| TEXAS INSTRUMENTS INCORPORATED
| Standard Linear and Logic Group
| IBIS Model of SN74AHCT16245
| 16-BIT BUS TRANSCEIVERS WITH 3-STATE OUTPUTS
| This file contains package information for the following:
|  SSOP 48-pin (DL) package as [Component] AHCT16245_DL
|  TSSOP 48-pin (DGG) package as [Component] AHCT16245_DGG
|  TVSOP 48-pin (DGV) package as [Component] AHCT16245_DGV
| This device can be powered at the following Vccs:
|  5 volt Vcc
| This file provides unique models under the [Model Selector] for each Vcc.
| For operation at a specific Vcc, select the appropriate model after each
| [Model Selector] keyword.
[IBIS Ver]   3.2
[Comment char]  |_char
[File Name]   sn74ahct16245.ibs
[File Rev]   1.1 | a_die
[Date]   January 15, 2001
[Source]   Data created from TI-SPICE simulations at TI-SLL.
[Notes]   The following is an IBIS list for the AHCT16245.
   Please contact sllibis@ti.com with questions and
   comments concerning SLL IBIS models.
[Disclaimer] Property of Texas Instruments Incorporated.  Unauthorized
   reproduction and/or distribution is strictly prohibited.
   This product is protected under copyright law.
   Created  2001, (C) Copyright  2001, Texas Instruments
   Incorporated, All Rights Reserved
   UNLESS THERE IS A SIGNED, WRITTEN AGREEMENT TO THE
   CONTRARY, TEXAS INSTRUMENTS (TI) IS PROVIDING THE IBIS
   MODELS  AND WITHOUT ANY WARRANTY, EXPRESSED OR
   IMPLIED.  TI assumes no liability for:
   1) the accuracy of the IBIS models provided to your
   company;
   2) the proper functioning of these IBIS Models in your
   design or for any resulting applications; or
   3) infringement of patents, copyrights or intellectual
   property rights resulting from your use of these IBIS
   models.
   TI provides IBIS Models as a service to our customers.
   You and your company shall not distribute, sell or give
   these models to anyone else without prior written
   permission from TI.
   TI reserves the right to make changes to our products or
   to discontinue any semiconductor product or service
   without notice, and advises our customers to obtain the
   latest version of relevant information to verify, before
   placing orders, that the information being relied on is
   current.
   Please be aware that your receipt and use of the IBIS
   information provided shall serve as acceptance of these
   terms and conditions.  If you do not accept these terms,
   you should return or destroy the IBIS models and any
   other accompanying information immediately.
| Component AHCT16245_DL 48-pin SSOP
[Component]   AHCT16245_DL
[Manufacturer]   Texas Instruments, Inc.
[Package]
|   typ   min   max
R_pkg   4.800e-02   3.800e-02   5.300e-02
L_pkg   6.046e-09   5.084e-09   7.968e-09
C_pkg   8.130e-13   5.690e-13   1.157e-12
[Pin]   signal_name   model_name   R_pin   L_pin   C_pin
1   1DIR   DIR   4.600e-02   7.968e-09   1.017e-12
2   1B1   AHCT16245_IO   4.400e-02   7.299e-09   1.157e-12
3   1B2   AHCT16245_IO   4.300e-02   6.765e-09   1.058e-12
4   GND   GND   4.100e-02   6.269e-09   9.330e-13
5   1B3   AHCT16245_IO   3.800e-02   5.856e-09   8.290e-13
6   1B4   AHCT16245_IO   4.600e-02   5.802e-09   7.900e-13
7   VCC   POWER   5.000e-02   5.656e-09   7.380e-13
8   1B5   AHCT16245_IO   5.300e-02   5.500e-09   6.430e-13
9   1B6   AHCT16245_IO   5.200e-02   5.304e-09   6.060e-13
10   GND   GND   5.300e-02   5.189e-09   5.830e-13
11   1B7   AHCT16245_IO   5.100e-02   5.084e-09   5.690e-13
12   1B8   AHCT16245_IO   5.300e-02   5.862e-09   8.330e-13
13   2B1   AHCT16245_IO   5.300e-02   5.862e-09   8.330e-13
14   2B2   AHCT16245_IO   5.100e-02   5.084e-09   5.690e-13
15   GND   GND   5.300e-02   5.189e-09   5.830e-13
16   2B3   AHCT16245_IO   5.200e-02   5.304e-09   6.060e-13
17   2B4   AHCT16245_IO   5.300e-02   5.500e-09   6.430e-13
18   VCC   POWER   5.000e-02   5.656e-09   7.380e-13
19   2B5   AHCT16245_IO   4.600e-02   5.802e-09   7.900e-13
20   2B6   AHCT16245_IO   3.800e-02   5.856e-09   8.290e-13
21   GND   GND   4.100e-02   6.269e-09   9.330e-13
22   2B7   AHCT16245_IO   4.300e-02   6.765e-09   1.058e-12
23   2B8   AHCT16245_IO   4.400e-02   7.299e-09   1.157e-12
24   2DIR   DIR   4.600e-02   7.968e-09   1.017e-12
25   2NOE   NOE   4.600e-02   7.968e-09   1.017e-12
26   2A8   AHCT16245_IO   4.400e-02   7.299e-09   1.157e-12
27   2A7   AHCT16245_IO   4.300e-02   6.765e-09   1.058e-12
28   GND   GND   4.100e-02   6.269e-09   9.330e-13
29   2A6   AHCT16245_IO   3.800e-02   5.856e-09   8.290e-13
30   2A5   AHCT16245_IO   4.600e-02   5.802e-09   7.900e-13
31   VCC   POWER   5.000e-02   5.656e-09   7.380e-13
32   2A4   AHCT16245_IO   5.300e-02   5.500e-09   6.430e-13
33   2A3   AHCT16245_IO   5.200e-02   5.304e-09   6.060e-13
34   GND   GND   5.300e-02   5.189e-09   5.830e-13
35   2A2   AHCT16245_IO   5.100e-02   5.084e-09   5.690e-13
36   2A1   AHCT16245_IO   5.300e-02   5.862e-09   8.330e-13
37   1A8   AHCT16245_IO   5.300e-02   5.862e-09   8.330e-13
38   1A7   AHCT16245_IO   5.100e-02   5.084e-09   5.690e-13
39   GND   GND   5.300e-02   5.189e-09   5.830e-13
40   1A6   AHCT16245_IO   5.200e-02   5.304e-09   6.060e-13
41   1A5   AHCT16245_IO   5.300e-02   5.500e-09   6.430e-13
42   VCC   POWER   5.000e-02   5.656e-09   7.380e-13
43   1A4   AHCT16245_IO   4.600e-02   5.802e-09   7.900e-13
44   1A3   AHCT16245_IO   3.800e-02   5.856e-09   8.290e-13
45   GND   GND   4.100e-02   6.269e-09   9.330e-13
46   1A2   AHCT16245_IO   4.300e-02   6.765e-09   1.058e-12
47   1A1   AHCT16245_IO   4.400e-02   7.299e-09   1.157e-12
48   1NOE   NOE   4.600e-02   7.967e-09   1.017e-12
| Component AHCT16245_DGG 48-pin TSSOP
[Component]   AHCT16245_DGG
[Manufacturer]   Texas Instruments, Inc.
[Package]
|   typ   min   max
R_pkg   6.200e-02   5.000e-02   7.800e-02
L_pkg   3.527e-09   3.128e-09   4.255e-09
C_pkg   5.300e-13   4.170e-13   6.850e-13
[Pin]   signal_name   model_name   R_pin   L_pin   C_pin
1   1DIR   DIR   5.000e-02   4.250e-09   6.710e-13
2   1B1   AHCT16245_IO   5.700e-02   3.956e-09   6.740e-13
3   1B2   AHCT16245_IO   7.100e-02   3.922e-09   6.190e-13
4   GND   GND   7.800e-02   3.841e-09   6.180e-13
5   1B3   AHCT16245_IO   5.600e-02   3.535e-09   5.550e-13
6   1B4   AHCT16245_IO   5.800e-02   3.464e-09   5.030e-13
7   VCC   POWER   6.000e-02   3.362e-09   4.980e-13
8   1B5   AHCT16245_IO   6.100e-02   3.293e-09   4.620e-13
9   1B6   AHCT16245_IO   6.300e-02   3.240e-09   4.550e-13
10   GND   GND   6.300e-02   3.175e-09   4.420e-13
11   1B7   AHCT16245_IO   6.400e-02   3.153e-09   4.290e-13
12   1B8   AHCT16245_IO   6.500e-02   3.128e-09   4.180e-13
13   2B1   AHCT16245_IO   6.500e-02   3.128e-09   4.180e-13
14   2B2   AHCT16245_IO   6.400e-02   3.154e-09   4.290e-13
15   GND   GND   6.300e-02   3.174e-09   4.420e-13
16   2B3   AHCT16245_IO   6.300e-02   3.241e-09   4.550e-13
17   2B4   AHCT16245_IO   6.100e-02   3.293e-09   4.620e-13
18   VCC   POWER   6.000e-02   3.362e-09   4.970e-13
19   2B5   AHCT16245_IO   5.800e-02   3.464e-09   5.030e-13
20   2B6   AHCT16245_IO   5.600e-02   3.537e-09   5.600e-13
21   GND   GND   7.700e-02   3.839e-09   6.260e-13
22   2B7   AHCT16245_IO   7.100e-02   3.917e-09   6.270e-13
23   2B8   AHCT16245_IO   5.800e-02   3.955e-09   6.850e-13
24   2DIR   DIR   5.200e-02   4.255e-09   6.790e-13
25   2NOE   NOE   5.100e-02   4.254e-09   6.760e-13
26   2A8   AHCT16245_IO   5.800e-02   3.957e-09   6.790e-13
27   2A7   AHCT16245_IO   7.100e-02   3.920e-09   6.210e-13
28   GND   GND   7.800e-02   3.843e-09   6.220e-13
29   2A6   AHCT16245_IO   5.600e-02   3.539e-09   5.600e-13
30   2A5   AHCT16245_IO   5.800e-02   3.466e-09   5.030e-13
31   VCC   POWER   6.000e-02   3.363e-09   4.970e-13
32   2A4   AHCT16245_IO   6.100e-02   3.294e-09   4.620e-13
33   2A3   AHCT16245_IO   6.300e-02   3.241e-09   4.540e-13
34   GND   GND   6.300e-02   3.175e-09   4.410e-13
35   2A2   AHCT16245_IO   6.400e-02   3.153e-09   4.290e-13
36   2A1   AHCT16245_IO   6.500e-02   3.129e-09   4.170e-13
37   1A8   AHCT16245_IO   6.500e-02   3.129e-09   4.170e-13
38   1A7   AHCT16245_IO   6.400e-02   3.152e-09   4.290e-13
39   GND   GND   6.400e-02   3.176e-09   4.410e-13
40   1A6   AHCT16245_IO   6.300e-02   3.241e-09   4.540e-13
41   1A5   AHCT16245_IO   6.100e-02   3.293e-09   4.620e-13
42   VCC   POWER   6.000e-02   3.363e-09   4.970e-13
43   1A4   AHCT16245_IO   5.800e-02   3.464e-09   5.030e-13
44   1A3   AHCT16245_IO   5.600e-02   3.534e-09   5.610e-13
45   GND   GND   7.800e-02   3.841e-09   6.260e-13
46   1A2   AHCT16245_IO   7.100e-02   3.920e-09   6.220e-13
47   1A1   AHCT16245_IO   5.700e-02   3.955e-09   6.770e-13
48   1NOE   NOE   5.100e-02   4.252e-09   6.720e-13
| Component AHCT16245_DGV 48-pin TVSOP
[Component]   AHCT16245_DGV
[Manufacturer]   Texas Instruments, Inc.
[Package]
|   typ   min   max
R_pkg   7.000e-02   4.900e-02   8.500e-02
L_pkg   3.013e-09   2.743e-09   3.408e-09
C_pkg   3.710e-13   2.940e-13   5.110e-13
[Pin]   signal_name   model_name   R_pin   L_pin   C_pin
1   1DIR   DIR   4.900e-02   3.393e-09   4.970e-13
2   1B1   AHCT16245_IO   6.000e-02   3.250e-09   5.020e-13
3   1B2   AHCT16245_IO   7.700e-02   3.310e-09   4.510e-13
4   GND   GND   8.500e-02   3.299e-09   4.040e-13
5   1B3   AHCT16245_IO   8.300e-02   3.136e-09   3.600e-13
6   1B4   AHCT16245_IO   7.700e-02   3.019e-09   3.630e-13
7   VCC   POWER   6.500e-02   2.882e-09   3.490e-13
8   1B5   AHCT16245_IO   6.600e-02   2.829e-09   3.140e-13
9   1B6   AHCT16245_IO   6.700e-02   2.796e-09   3.140e-13
10   GND   GND   6.900e-02   2.754e-09   3.080e-13
11   1B7   AHCT16245_IO   7.000e-02   2.753e-09   3.010e-13
12   1B8   AHCT16245_IO   7.100e-02   2.745e-09   2.940e-13
13   2B1   AHCT16245_IO   7.000e-02   2.744e-09   2.940e-13
14   2B2   AHCT16245_IO   7.000e-02   2.754e-09   3.010e-13
15   GND   GND   6.900e-02   2.754e-09   3.080e-13
16   2B3   AHCT16245_IO   6.700e-02   2.796e-09   3.140e-13
17   2B4   AHCT16245_IO   6.600e-02   2.829e-09   3.140e-13
18   VCC   POWER   6.500e-02   2.883e-09   3.500e-13
19   2B5   AHCT16245_IO   7.500e-02   3.014e-09   3.630e-13
20   2B6   AHCT16245_IO   8.000e-02   3.128e-09   3.580e-13
21   GND   GND   8.400e-02   3.295e-09   4.030e-13
22   2B7   AHCT16245_IO   7.800e-02   3.311e-09   4.520e-13
23   2B8   AHCT16245_IO   6.200e-02   3.259e-09   5.010e-13
24   2DIR   DIR   5.200e-02   3.404e-09   4.960e-13
25   2NOE   NOE   5.300e-02   3.397e-09   5.050e-13
26   2A8   AHCT16245_IO   6.200e-02   3.249e-09   5.110e-13
27   2A7   AHCT16245_IO   7.700e-02   3.308e-09   4.530e-13
28   GND   GND   8.200e-02   3.289e-09   4.030e-13
29   2A6   AHCT16245_IO   7.800e-02   3.121e-09   3.590e-13
30   2A5   AHCT16245_IO   7.400e-02   3.010e-09   3.630e-13
31   VCC   POWER   6.500e-02   2.883e-09   3.490e-13
32   2A4   AHCT16245_IO   6.700e-02   2.829e-09   3.140e-13
33   2A3   AHCT16245_IO   6.700e-02   2.795e-09   3.140e-13
34   GND   GND   6.900e-02   2.753e-09   3.070e-13
35   2A2   AHCT16245_IO   7.000e-02   2.753e-09   3.010e-13
36   2A1   AHCT16245_IO   7.000e-02   2.743e-09   2.940e-13
37   1A8   AHCT16245_IO   7.000e-02   2.743e-09   2.940e-13
38   1A7   AHCT16245_IO   7.000e-02   2.753e-09   3.010e-13
39   GND   GND   6.900e-02   2.754e-09   3.070e-13
40   1A6   AHCT16245_IO   6.800e-02   2.797e-09   3.140e-13
41   1A5   AHCT16245_IO   6.700e-02   2.830e-09   3.140e-13
42   VCC   POWER   6.400e-02   2.880e-09   3.490e-13
43   1A4   AHCT16245_IO   7.200e-02   3.004e-09   3.620e-13
44   1A3   AHCT16245_IO   7.800e-02   3.121e-09   3.590e-13
45   GND   GND   8.400e-02   3.296e-09   4.030e-13
46   1A2   AHCT16245_IO   7.700e-02   3.308e-09   4.510e-13
47   1A1   AHCT16245_IO   6.200e-02   3.258e-09   4.990e-13
48   1NOE   NOE   5.300e-02   3.408e-09   4.940e-13
| Models and submodels in the file (3): NOE (Input), DIR (Input), AHCT16245_IO (I/O)
